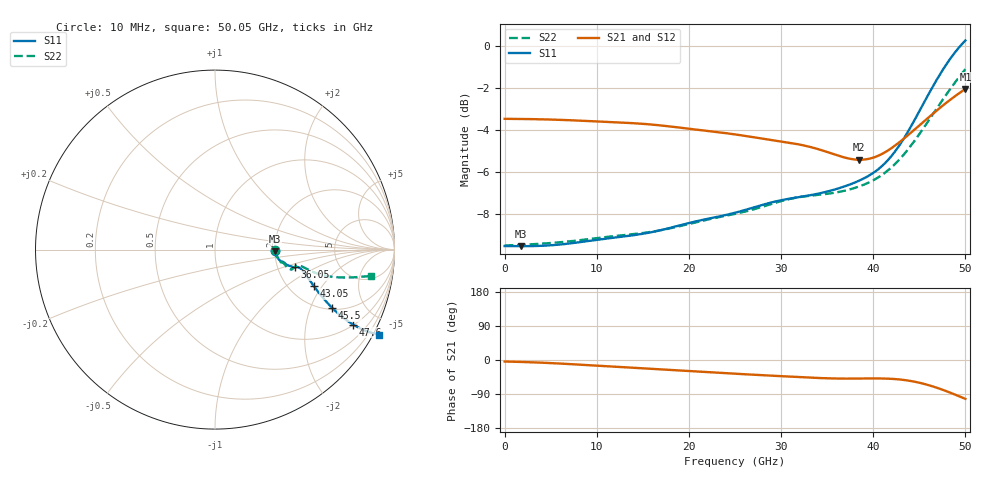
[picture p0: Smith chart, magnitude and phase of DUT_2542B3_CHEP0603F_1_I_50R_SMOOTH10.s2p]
! Touchstone file from project
! Exported from ElectronicsDesktop 2025.1.3
# GHz S MA R 50.000000
! Terminal data exported
! Port[1] = Port1
! Port[2] = Port2
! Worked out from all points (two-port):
!   144 points, 10 MHz to 50.05 GHz, reference 50 ohm
!   highest |S21| = -2.06 dB at 50.05 GHz (marker M1); lowest = -5.4 dB at 38.5 GHz (marker M2)
!   |S21| within 3 dB of the highest: start of sweep to 34.99 GHz; 41.39 GHz to end of sweep
!   lowest |S11| = -9.6 dB at 1.76 GHz (marker M3), VSWR 2.00, Z = 99.8 - j1.95 ohm
!   |S11| at or under -10 dB: nowhere
!   |S22| runs from -9.5 to -1.1 dB; largest |S21 - S12| = 0.0092
!   S11 on the Smith chart (normalised r, x): 10 MHz: 2.00, -0.02; 36.05 GHz: 2.49, -0.62; 43.05 GHz: 2.70, -1.67; 45.5 GHz: 2.08, -2.87; 47.6 GHz: 1.02, -3.68; 50.05 GHz: -0.26, -4.09
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0.01  0.3331 -0.9  0.6698 -4.0  0.6696 -4.0  0.3341 -0.8
! Gamma 0 0 0 0
! Port Impedance 50 0 50 0
1.75975  0.3328 -1.5  0.6693 -5.1  0.6689 -5.0  0.3353 -1.3
4.9093  0.3343 -3.3  0.6673 -8.0  0.6664 -7.9  0.3385 -3.1
8.4088  0.3408 -5.6  0.6628 -12.6  0.6613 -12.5  0.3444 -5.8
13.3081  0.3518 -7.3  0.6552 -19.6  0.6534 -19.5  0.3544 -7.8
16.8076  0.3627 -9.2  0.6465 -24.7  0.6453 -24.5  0.3627 -9.9
25.2064  0.4008 -11.4  0.6141 -36.4  0.6143 -36.1  0.3982 -12.2
29.75575  0.427 -12.2  0.5928 -42.3  0.5931 -42.0  0.4245 -14.3
33.6052  0.4421 -12.6  0.5708 -47.0  0.571 -46.6  0.4401 -14.6
36.05485  0.4556 -12.4  0.5488 -48.9  0.5487 -48.5  0.4472 -13.6
38.5045  0.4768 -12.0  0.535 -48.9  0.5345 -48.5  0.4618 -11.4
40.25425  0.5014 -13.4  0.5432 -48.6  0.5424 -48.2  0.4808 -10.7
42.004  0.5453 -17.2  0.5698 -49.7  0.5687 -49.2  0.5127 -11.6
43.05385  0.5864 -20.2  0.593 -51.8  0.5917 -51.3  0.5408 -12.4
43.75375  0.6209 -22.2  0.6105 -53.9  0.6091 -53.4  0.5639 -12.9
44.45365  0.6607 -24.1  0.6293 -56.9  0.6278 -56.3  0.5904 -13.2
45.5035  0.7287 -26.4  0.659 -62.6  0.6574 -62.1  0.6364 -13.3
46.55335  0.8025 -27.9  0.6897 -70.0  0.6879 -69.4  0.6884 -12.9
47.6032  0.8769 -28.5  0.7205 -78.8  0.7186 -78.2  0.7446 -12.1
48.3031  0.9247 -28.5  0.7408 -85.2  0.7389 -84.6  0.7832 -11.4
49.003  0.9696 -28.2  0.7606 -92.0  0.7587 -91.3  0.8222 -10.7
50.05285  1.03 -27.4  0.7892 -102.6  0.7872 -101.9  0.8799 -9.6
